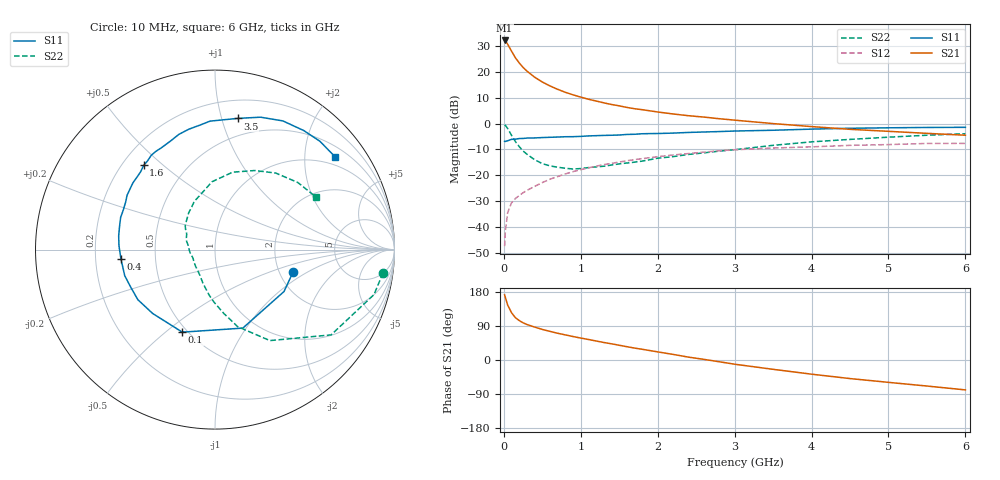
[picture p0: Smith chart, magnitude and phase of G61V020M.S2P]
! SIEMENS Small Signal Semiconductors
! BFG193
! Si NPN RF Bipolar Junction Transistor in SOT223
! VCE = 1 V  IC = 20 mA
! Common Emitter S-Parameters:  August  1996
# GHz  S  MA  R  50
!  f  S11  S21  S12  S22
! GHz  MAG  ANG  MAG  ANG  MAG  ANG  MAG  ANG
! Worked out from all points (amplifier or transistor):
!   36 points, 10 MHz to 6 GHz, reference 50 ohm
!   highest |S21| = 32.2 dB at 10 MHz (marker M1)
!   |S21| within 3 dB of that: start of sweep to 78.51 MHz
!   unconditionally stable (mu >= 1): 619.9 MHz to 2.919 GHz; 3.377 GHz to 3.548 GHz
!   at 250 MHz: K = 0.76, MSG = 24.3 dB, |S12| = -26.8 dB
!   at 1.4 GHz: K = 1.07, MAG = 9.8 dB, |S12| = -15.4 dB
!   at 6 GHz: K = 0.96, MSG = 1.6 dB, |S12| = -7.7 dB
!   S11 on the Smith chart (normalised r, x): 10 MHz: 2.37, -0.76; 100 MHz: 0.47, -0.57; 400 MHz: 0.31, -0.04; 1.6 GHz: 0.29, +0.43; 3.5 GHz: 0.35, +1.13; 6 GHz: 0.75, +2.74
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0.01  0.4524 -16.3  40.82 172.0  0.0042 83.5  0.9451 -7.9
0.02  0.4498 -31.3  39.89 165.0  0.0083 78.8  0.9207 -15.8
0.05  0.464 -70.5  34.49 144.8  0.0188 67.5  0.8026 -36.3
0.1  0.4947 -111.6  25.29 124.8  0.0291 56.5  0.5921 -58.9
0.15  0.4973 -134.3  18.87 111.6  0.0352 52.8  0.4475 -73.6
0.2  0.5125 -147.0  14.99 104.1  0.0402 53.1  0.3578 -82.3
0.25  0.5146 -156.7  12.26 98.2  0.0456 53.6  0.2938 -90.9
0.3  0.5235 -163.9  10.39 93.7  0.0506 55.0  0.2547 -97.5
0.4  0.5266 -174.3  7.931 86.9  0.0605 56.0  0.1994 -109.6
0.5  0.5354 177.8  6.382 80.7  0.0718 56.2  0.1671 -120.1
0.6  0.542 171.9  5.357 75.5  0.0835 56.4  0.1512 -129.6
0.7  0.5476 166.1  4.612 70.6  0.094 55.8  0.1424 -139.6
0.9  0.5567 156.5  3.602 61.9  0.1171 53.2  0.1316 -158.5
1.1  0.5759 148.3  2.962 54.1  0.1382 50.2  0.1402 -172.9
1.3  0.5895 140.8  2.521 46.2  0.1601 46.3  0.1491 172.5
1.6  0.6151 130.2  2.054 35.1  0.1902 39.8  0.172 158.0
2.2  0.6533 112.4  1.534 14.8  0.246 26.1  0.2281 133.8
3  0.7163 92.2  1.164 -11.1  0.3108 7.5  0.311 106.4
3.5  0.7418 80.2  0.999 -24.6  0.3354 -5.4  0.3785 92.5
4.5  0.8106 62.2  0.773 -49.0  0.3781 -24.7  0.4932 63.3
5.5  0.8403 45.9  0.646 -68.7  0.4117 -47.0  0.5939 39.0
6  0.8452 37.8  0.594 -78.9  0.4122 -59.7  0.6351 27.4
